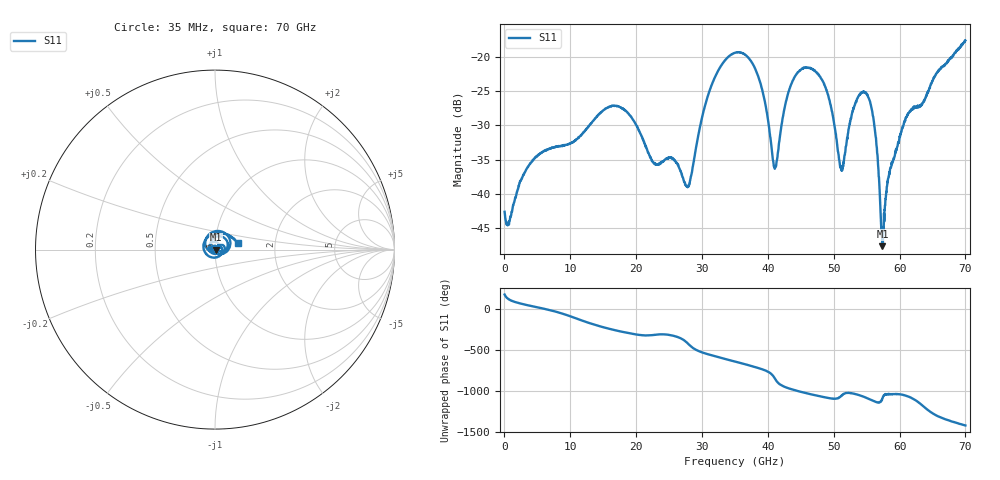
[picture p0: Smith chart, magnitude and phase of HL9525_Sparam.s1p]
! 4/11/2024 8:06:19 AM
! CHANNEL.1
! TR.MEASUREMENT
! CORRECTED.DATA
# GHZ S RI R 50.0
! FREQ.GHZ  S11RE  S11IM
!; PortSelection: Port_1
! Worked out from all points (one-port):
!   2000 points, 35 MHz to 70 GHz, reference 50 ohm
!   lowest |S11| = -47.6 dB at 57.4 GHz (marker M1), VSWR 1.01, Z = 50.4 - j0.0954 ohm
!   |S11| at or under -10 dB: start of sweep to end of sweep
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0.035  -0.00735 0.00115
0.665  -0.00256 0.00557
2.52  0.00626 0.0109
4.305  0.0156 0.00828
8.785  0.011 -0.0196
17.535  0.00481 0.0426
22.68  0.013 0.0106
26.285  0.016 0.00401
27.93  0.00373 -0.0107
31.255  -0.0532 0.0239
35.035  0.0292 0.1026
38.465  0.0735 -0.0023
41.09  -0.0107 -0.0111
42.595  -0.025 0.0354
43.785  -0.00355 0.067
45.815  0.0539 0.0632
48.16  0.068 0.00893
49.525  0.0436 -0.0102
51.17  0.0145 0.00484
52.535  0.0215 0.0264
54.11  0.0508 0.0174
55.475  0.0428 -0.0203
56.35  0.0153 -0.0223
57.4  0.00407 -0.000947
58.52  0.0115 0.00895
61.285  0.0381 0.00638
65.205  -0.0633 0.0293
70  0.1256 0.0366
